
DATA_BLOCK DB3450
TITLE=
VERSION : 0.1

STRUCT
   CM_ID : STRING  [8 ] := '=PRM'; //COMPOSITE MACHINE
   STATION_ID : STRING  [8 ] := '++OP10'; //STATION - TRATTO - ZONE
   ELEMENT_ID : STRING  [8 ] := '@'; //+80FTR903
   DB_ID : INT := 1 ; //DB SIZE OR TYPE
   PART_STYLE : STRING  [12 ]; //PART STYLE ON LAST STATION
   ACT_CYCLE_TIME : INT ; //ACTUAL CYCLE TIME FOR THIS STYLE
   COUNT_GOOD : INT ; //COUNTER GOOD PIECES
   COUNT_SCRAP : INT ; //COUNTER SCRAP PIECES
   SPARE_00 : ARRAY  [0 .. 15 ] OF //SPARE INTEGER
   INT ;
   SPARE_01 : ARRAY  [0 .. 17 ] OF //SPARE INTEGER
   INT ;
   CODE_EVENT : ARRAY  [0 .. 7 ] OF //CODE EVENT - EXTENDED FAULT CODE DIAGNOSTIC
   INT ;
   EVENT : STRUCT
E0000 : BOOL ; //+80FTR903-M1; MS. SERRANDA OK;58

E0001 : BOOL ; //+80FTR903-M1; MS. APERTO;58

E0002 : BOOL ; //+80FTR903-M1; MS. CHIUSO;58

E0003 : BOOL ; //+80FTR903-M1;MS.GENERALI ERRORE;1

E0004 : BOOL ; //+80FTR903-M1; MS. MS_04;58

E0005 : BOOL ; //+80FTR903-M1; MS. MS_05;58

E0006 : BOOL ; //+80FTR903-M1; MS. MS_06;58

E0007 : BOOL ; //+80FTR903-M1; MS. MS_07;58

E0008 : BOOL ; //+80FTR903-M1; MS. MS_10;58

E0009 : BOOL ; //+80FTR903-M1; MS. MS_11;58

E0010 : BOOL ; //+80FTR903-M1; MS. MS_12;58

E0011 : BOOL ; //+80FTR903-M1; MS. MS_13;58

E0012 : BOOL ; //+80FTR903-M1; MS. MS_14;58

E0013 : BOOL ; //+80FTR903-M1; MS. MS_15;58

E0014 : BOOL ; //+80FTR903-M1; MS. MS_16;58

E0015 : BOOL ; //+80FTR903-M1; MS. MS_17;58

E0016 : BOOL ; //+80FTR903-M1; ME. DURATA APERTO;1

E0017 : BOOL ; //+80FTR903-M1; ME. DURATA CHIUDI;1

E0018 : BOOL ; //+80FTR903-M1; ME. PLAUSIBILITA;1

E0019 : BOOL ; //+80FTR903-M1; ME. FILO ROTTURA;1

E0020 : BOOL ; //+80FTR903-M1; ME. ME_04;58

E0021 : BOOL ; //+80FTR903-M1; ME. ME_05;58

E0022 : BOOL ; //+80FTR903-M1; ME. ME_06;58

E0023 : BOOL ; //+80FTR903-M1; ME. ME_07;58

E0024 : BOOL ; //+80FTR903-M1; ME. ME_10;58

E0025 : BOOL ; //+80FTR903-M1; ME. ME_11;58

E0026 : BOOL ; //+80FTR903-M1; ME. ME_12;58

E0027 : BOOL ; //+80FTR903-M1; ME. ME_13;58

E0028 : BOOL ; //+80FTR903-M1; ME. ME_14;58

E0029 : BOOL ; //+80FTR903-M1; ME. ME_15;58

E0030 : BOOL ; //+80FTR903-M1; ME. ME_16;58

E0031 : BOOL ; //+80FTR903-M1; ME. ME_17;58

E0032 : BOOL ; //+80FTR903-Y1_1; MS. APERTO;58

E0033 : BOOL ; //+80FTR903-Y1_1; MS. CHIUSO;58

E0034 : BOOL ; //+80FTR903-Y1_1;MS.GENERALI ERRORE;1

E0035 : BOOL ; //+80FTR903-Y1_1;MS.GENERALI AVVERTIMENTO;2

E0036 : BOOL ; //+80FTR903-Y1_1; MS. MS_04;58

E0037 : BOOL ; //+80FTR903-Y1_1; MS. MS_05;58

E0038 : BOOL ; //+80FTR903-Y1_1; MS. MS_06;58

E0039 : BOOL ; //+80FTR903-Y1_1; MS. MS_07;58

E0040 : BOOL ; //+80FTR903-Y1_1; MS. MS_10;58

E0041 : BOOL ; //+80FTR903-Y1_1; MS. MS_11;58

E0042 : BOOL ; //+80FTR903-Y1_1; MS. MS_12;58

E0043 : BOOL ; //+80FTR903-Y1_1; MS. MS_13;58

E0044 : BOOL ; //+80FTR903-Y1_1; MS. MS_14;58

E0045 : BOOL ; //+80FTR903-Y1_1; MS. MS_15;58

E0046 : BOOL ; //+80FTR903-Y1_1; MS. MS_16;58

E0047 : BOOL ; //+80FTR903-Y1_1; MS. MS_17;58

E0048 : BOOL ; //+80FTR903-Y1_1; ME. DURATA APERTO;1

E0049 : BOOL ; //+80FTR903-Y1_1; ME. DURATA CHIUDI;1

E0050 : BOOL ; //+80FTR903-Y1_1; ME. PLAUSIBILITA;1

E0051 : BOOL ; //+80FTR903-Y1_1; ME. FILO ROTTURA;1

E0052 : BOOL ; //+80FTR903-Y1_1; ME. PERSO POSIZIONE APERTO;2

E0053 : BOOL ; //+80FTR903-Y1_1; ME. PERSO POSIZIONE CHIUSA;2

E0054 : BOOL ; //+80FTR903-Y1_1; ME. ME_06;58

E0055 : BOOL ; //+80FTR903-Y1_1; ME. ME_07;58

E0056 : BOOL ; //+80FTR903-Y1_1; ME. ME_10;58

E0057 : BOOL ; //+80FTR903-Y1_1; ME. ME_11;58

E0058 : BOOL ; //+80FTR903-Y1_1; ME. ME_12;58

E0059 : BOOL ; //+80FTR903-Y1_1; ME. ME_13;58

E0060 : BOOL ; //+80FTR903-Y1_1; ME. ME_14;58

E0061 : BOOL ; //+80FTR903-Y1_1; ME. ME_15;58

E0062 : BOOL ; //+80FTR903-Y1_1; ME. ME_16;58

E0063 : BOOL ; //+80FTR903-Y1_1; ME. ME_17;58

E0064 : BOOL ; //+80FTR903-Y1_2; MS. APERTO;58

E0065 : BOOL ; //+80FTR903-Y1_2; MS. CHIUSO;58

E0066 : BOOL ; //+80FTR903-Y1_2;MS.GENERALI ERRORE;1

E0067 : BOOL ; //+80FTR903-Y1_2;MS.GENERALI AVVERTIMENTO;2

E0068 : BOOL ; //+80FTR903-Y1_2; MS. MS_04;58

E0069 : BOOL ; //+80FTR903-Y1_2; MS. MS_05;58

E0070 : BOOL ; //+80FTR903-Y1_2; MS. MS_06;58

E0071 : BOOL ; //+80FTR903-Y1_2; MS. MS_07;58

E0072 : BOOL ; //+80FTR903-Y1_2; MS. MS_10;58

E0073 : BOOL ; //+80FTR903-Y1_2; MS. MS_11;58

E0074 : BOOL ; //+80FTR903-Y1_2; MS. MS_12;58

E0075 : BOOL ; //+80FTR903-Y1_2; MS. MS_13;58

E0076 : BOOL ; //+80FTR903-Y1_2; MS. MS_14;58

E0077 : BOOL ; //+80FTR903-Y1_2; MS. MS_15;58

E0078 : BOOL ; //+80FTR903-Y1_2; MS. MS_16;58

E0079 : BOOL ; //+80FTR903-Y1_2; MS. MS_17;58

E0080 : BOOL ; //+80FTR903-Y1_2; ME. DURATA APERTO;1

E0081 : BOOL ; //+80FTR903-Y1_2; ME. DURATA CHIUDI;1

E0082 : BOOL ; //+80FTR903-Y1_2; ME. PLAUSIBILITA;1

E0083 : BOOL ; //+80FTR903-Y1_2; ME. FILO ROTTURA;1

E0084 : BOOL ; //+80FTR903-Y1_2; ME. PERSO POSIZIONE APERTO;2

E0085 : BOOL ; //+80FTR903-Y1_2; ME. PERSO POSIZIONE CHIUSA;2

E0086 : BOOL ; //+80FTR903-Y1_2; ME. ME_06;58

E0087 : BOOL ; //+80FTR903-Y1_2; ME. ME_07;58

E0088 : BOOL ; //+80FTR903-Y1_2; ME. ME_10;58

E0089 : BOOL ; //+80FTR903-Y1_2; ME. ME_11;58

E0090 : BOOL ; //+80FTR903-Y1_2; ME. ME_12;58

E0091 : BOOL ; //+80FTR903-Y1_2; ME. ME_13;58

E0092 : BOOL ; //+80FTR903-Y1_2; ME. ME_14;58

E0093 : BOOL ; //+80FTR903-Y1_2; ME. ME_15;58

E0094 : BOOL ; //+80FTR903-Y1_2; ME. ME_16;58

E0095 : BOOL ; //+80FTR903-Y1_2; ME. ME_17;58

E0096 : BOOL ; //+80FTR903-Y1_3; MS. APERTO;58

E0097 : BOOL ; //+80FTR903-Y1_3; MS. CHIUSO;58

E0098 : BOOL ; //+80FTR903-Y1_3;MS.GENERALI ERRORE;1

E0099 : BOOL ; //+80FTR903-Y1_3;MS.GENERALI AVVERTIMENTO;2

E0100 : BOOL ; //+80FTR903-Y1_3; MS. MS_04;58

E0101 : BOOL ; //+80FTR903-Y1_3; MS. MS_05;58

E0102 : BOOL ; //+80FTR903-Y1_3; MS. MS_06;58

E0103 : BOOL ; //+80FTR903-Y1_3; MS. MS_07;58

E0104 : BOOL ; //+80FTR903-Y1_3; MS. MS_10;58

E0105 : BOOL ; //+80FTR903-Y1_3; MS. MS_11;58

E0106 : BOOL ; //+80FTR903-Y1_3; MS. MS_12;58

E0107 : BOOL ; //+80FTR903-Y1_3; MS. MS_13;58

E0108 : BOOL ; //+80FTR903-Y1_3; MS. MS_14;58

E0109 : BOOL ; //+80FTR903-Y1_3; MS. MS_15;58

E0110 : BOOL ; //+80FTR903-Y1_3; MS. MS_16;58

E0111 : BOOL ; //+80FTR903-Y1_3; MS. MS_17;58

E0112 : BOOL ; //+80FTR903-Y1_3; ME. DURATA APERTO;1

E0113 : BOOL ; //+80FTR903-Y1_3; ME. DURATA CHIUDI;1

E0114 : BOOL ; //+80FTR903-Y1_3; ME. PLAUSIBILITA;1

E0115 : BOOL ; //+80FTR903-Y1_3; ME. FILO ROTTURA;1

E0116 : BOOL ; //+80FTR903-Y1_3; ME. PERSO POSIZIONE APERTO;2

E0117 : BOOL ; //+80FTR903-Y1_3; ME. PERSO POSIZIONE CHIUSA;2

E0118 : BOOL ; //+80FTR903-Y1_3; ME. ME_06;58

E0119 : BOOL ; //+80FTR903-Y1_3; ME. ME_07;58

E0120 : BOOL ; //+80FTR903-Y1_3; ME. ME_10;58

E0121 : BOOL ; //+80FTR903-Y1_3; ME. ME_11;58

E0122 : BOOL ; //+80FTR903-Y1_3; ME. ME_12;58

E0123 : BOOL ; //+80FTR903-Y1_3; ME. ME_13;58

E0124 : BOOL ; //+80FTR903-Y1_3; ME. ME_14;58

E0125 : BOOL ; //+80FTR903-Y1_3; ME. ME_15;58

E0126 : BOOL ; //+80FTR903-Y1_3; ME. ME_16;58

E0127 : BOOL ; //+80FTR903-Y1_3; ME. ME_17;58

E0128 : BOOL ; //+80FTR903-A1; MS. DISPLAY RILASCIATO;58

E0129 : BOOL ; //+80FTR903-A1; MS. MS_01;58

E0130 : BOOL ; //+80FTR903-A1; MS. MS_02;58

E0131 : BOOL ; //+80FTR903-A1; MS. MS_03;58

E0132 : BOOL ; //+80FTR903-A1; MS. MS_04;58

E0133 : BOOL ; //+80FTR903-A1; MS. MS_05;58

E0134 : BOOL ; //+80FTR903-A1; MS. MS_06;58

E0135 : BOOL ; //+80FTR903-A1; MS. MS_07;58

E0136 : BOOL ; //+80FTR903-A1; MS. MS_10;58

E0137 : BOOL ; //+80FTR903-A1; MS. MS_11;58

E0138 : BOOL ; //+80FTR903-A1; MS. MS_12;58

E0139 : BOOL ; //+80FTR903-A1; MS. MS_13;58

E0140 : BOOL ; //+80FTR903-A1; MS. MS_14;58

E0141 : BOOL ; //+80FTR903-A1; MS. MS_15;58

E0142 : BOOL ; //+80FTR903-A1; MS. MS_16;58

E0143 : BOOL ; //+80FTR903-A1; MS. MS_17;58

E0144 : BOOL ; //+80FTR903-A1; ME. ME_00;58

E0145 : BOOL ; //+80FTR903-A1; ME. ME_01;58

E0146 : BOOL ; //+80FTR903-A1; ME. ME_02;58

E0147 : BOOL ; //+80FTR903-A1; ME. ME_03;58

E0148 : BOOL ; //+80FTR903-A1; ME. ME_04;58

E0149 : BOOL ; //+80FTR903-A1; ME. ME_05;58

E0150 : BOOL ; //+80FTR903-A1; ME. ME_06;58

E0151 : BOOL ; //+80FTR903-A1; ME. ME_07;58

E0152 : BOOL ; //+80FTR903-A1; ME. ME_10;58

E0153 : BOOL ; //+80FTR903-A1; ME. ME_11;58

E0154 : BOOL ; //+80FTR903-A1; ME. ME_12;58

E0155 : BOOL ; //+80FTR903-A1; ME. ME_13;58

E0156 : BOOL ; //+80FTR903-A1; ME. ME_14;58

E0157 : BOOL ; //+80FTR903-A1; ME. ME_15;58

E0158 : BOOL ; //+80FTR903-A1; ME. ME_16;58

E0159 : BOOL ; //+80FTR903-A1; ME. ME_17;58

E0160 : BOOL ; //+80FTR903-A2;MS.MODO AUTOMATICO;19

E0161 : BOOL ; //+80FTR903-A2;MS.MODALITA MANUALE;16

E0162 : BOOL ; //+80FTR903-A2; MS. ECUBE A DISPOSIZIONE;58

E0163 : BOOL ; //+80FTR903-A2; MS. ECUBE NON DISPONIBILE;58

E0164 : BOOL ; //+80FTR903-A2; MS. ECUBE BLOCCATO;58

E0165 : BOOL ; //+80FTR903-A2; MS. ECUBE SBLOCCATO;58

E0166 : BOOL ; //+80FTR903-A2; MS. ECUBE ATTRACCO;58

E0167 : BOOL ; //+80FTR903-A2; MS. ECUBE ATTRACCATO;58

E0168 : BOOL ; //+80FTR903-A2; MS. ECUBE SGANCIO;58

E0169 : BOOL ; //+80FTR903-A2; MS. ECUBE SGANCIATO;58

E0170 : BOOL ; //+80FTR903-A2; MS. STAMPA ERRORE;58

E0171 : BOOL ; //+80FTR903-A2; MS. AVVIO PRODUZIONE;19

E0172 : BOOL ; //+80FTR903-A2; MS. PRODUZIONE PRONTO;19

E0173 : BOOL ; //+80FTR903-A2;MS.GENERALI ERRORE;1

E0174 : BOOL ; //+80FTR903-A2;MS.GENERALI AVVERTIMENTO;2

E0175 : BOOL ; //+80FTR903-A2;MS.RILASCIO;17

E0176 : BOOL ; //+80FTR903-A2; ME. ECUBE TIPO SBAGLIATO;1

E0177 : BOOL ; //+80FTR903-A2; ME. COMUNICAZIONE TIMEOUT;1

E0178 : BOOL ; //+80FTR903-A2; ME. SEGNALE RFID PERSO;1

E0179 : BOOL ; //+80FTR903-A2; ME. ATTRACCATO IMPOSSIBILE;1

E0180 : BOOL ; //+80FTR903-A2; ME. SGANCIATO IMPOSSIBLE;1

E0181 : BOOL ; //+80FTR903-A2; ME. ATTRACCATO FALLITO;1

E0182 : BOOL ; //+80FTR903-A2; ME. SGANCIATO FALLITO;1

E0183 : BOOL ; //+80FTR903-A2; ME. SOSTITUIRE TEMPO SCADUTO;2

E0184 : BOOL ; //+80FTR903-A2; ME. ME_10;58

E0185 : BOOL ; //+80FTR903-A2; ME. ME_11;58

E0186 : BOOL ; //+80FTR903-A2; ME. ME_12;58

E0187 : BOOL ; //+80FTR903-A2; ME. ME_13;58

E0188 : BOOL ; //+80FTR903-A2; ME. ME_14;58

E0189 : BOOL ; //+80FTR903-A2; ME. ME_15;58

E0190 : BOOL ; //+80FTR903-A2; ME. ME_16;58

E0191 : BOOL ; //+80FTR903-A2; ME. ME_17;58

E0192 : BOOL ; //+80FTR903-A3; MS. ORIFICE SENSORE DI PRESSIONE OK;58

E0193 : BOOL ; //+80FTR903-A3; MS. ORIFICE ERRORE GENERALE;1

E0194 : BOOL ; //+80FTR903-A3; MS. ORIFICE AVVERTENZE GENERALE;2

E0195 : BOOL ; //+80FTR903-A3; MS. ECUBE SENSORE DI PRESSIONE OK;58

E0196 : BOOL ; //+80FTR903-A3; MS. ECUBE ERRORE GENERALE;1

E0197 : BOOL ; //+80FTR903-A3; MS. ECEBU AVVERTENZE GENERALE;2

E0198 : BOOL ; //+80FTR903-A3; MS. 2FILTER SENSORE DI PRESSIONE OK;58

E0199 : BOOL ; //+80FTR903-A3; MS. 2FILTER ERRORE GENERALE;1

E0200 : BOOL ; //+80FTR903-A3; MS. 2FILTER AVVERTENZE GENERALE;2

E0201 : BOOL ; //+80FTR903-A3; MS. MS_11;58

E0202 : BOOL ; //+80FTR903-A3; MS. MS_12;58

E0203 : BOOL ; //+80FTR903-A3; MS. MS_13;58

E0204 : BOOL ; //+80FTR903-A3; MS. MS_14;58

E0205 : BOOL ; //+80FTR903-A3; MS. MS_15;58

E0206 : BOOL ; //+80FTR903-A3; MS. MS_16;58

E0207 : BOOL ; //+80FTR903-A3; MS. MS_17;58

E0208 : BOOL ; //+80FTR903-A3; ME. ORIFICE SONDA NON OK;1

E0209 : BOOL ; //+80FTR903-A3; ME. ORIFICE_H;2

E0210 : BOOL ; //+80FTR903-A3; ME. ORIFICE_HH;1

E0211 : BOOL ; //+80FTR903-A3; ME. ECUBE SONDA NON OK;1

E0212 : BOOL ; //+80FTR903-A3; ME. RIEMPIRE LIVELLO ECUBE_H;2

E0213 : BOOL ; //+80FTR903-A3; ME. RIEMPIRE LIVELLO ECUBE_HH;1

E0214 : BOOL ; //+80FTR903-A3; ME. 2FILTER SONDA NON OK;1

E0215 : BOOL ; //+80FTR903-A3; ME. RIEMPIRE LIVELLO 2FILTER_H;2

E0216 : BOOL ; //+80FTR903-A3; ME. RIEMPIRE LIVELLO 2FILTER_HH;1

E0217 : BOOL ; //+80FTR903-A3; ME. ME_11;58

E0218 : BOOL ; //+80FTR903-A3; ME. ME_12;58

E0219 : BOOL ; //+80FTR903-A3; ME. ME_13;58

E0220 : BOOL ; //+80FTR903-A3; ME. ME_14;58

E0221 : BOOL ; //+80FTR903-A3; ME. ME_15;58

E0222 : BOOL ; //+80FTR903-A3; ME. ME_16;58

E0223 : BOOL ; //+80FTR903-A3; ME. ME_17;58
E0224 : BOOL ;
E0225 : BOOL ;
E0226 : BOOL ;
E0227 : BOOL ;
E0228 : BOOL ;
E0229 : BOOL ;
E0230 : BOOL ;
E0231 : BOOL ;
E0232 : BOOL ;
E0233 : BOOL ;
E0234 : BOOL ;
E0235 : BOOL ;
E0236 : BOOL ;
E0237 : BOOL ;
E0238 : BOOL ;
E0239 : BOOL ;
E0240 : BOOL ;
E0241 : BOOL ;
E0242 : BOOL ;
E0243 : BOOL ;
E0244 : BOOL ;
E0245 : BOOL ;
E0246 : BOOL ;
E0247 : BOOL ;
E0248 : BOOL ;
E0249 : BOOL ;
E0250 : BOOL ;
E0251 : BOOL ;
E0252 : BOOL ;
E0253 : BOOL ;
E0254 : BOOL ;
E0255 : BOOL ;
END_STRUCT;
END_STRUCT;
BEGIN
CM_ID := '=PRM';
STATION_ID := '++OP10';
ELEMENT_ID := '@';
DB_ID := 1 ;
PART_STYLE := '';
ACT_CYCLE_TIME := 0;
COUNT_GOOD := 0;
COUNT_SCRAP := 0;
SPARE_00[0] := 0;
SPARE_00[1] := 0;
SPARE_00[2] := 0;
SPARE_00[3] := 0;
SPARE_00[4] := 0;
SPARE_00[5] := 0;
SPARE_00[6] := 0;
SPARE_00[7] := 0;
SPARE_00[8] := 0;
SPARE_00[9] := 0;
SPARE_00[10] := 0;
SPARE_00[11] := 0;
SPARE_00[12] := 0;
SPARE_00[13] := 0;
SPARE_00[14] := 0;
SPARE_00[15] := 0;
SPARE_01[0] := 0;
SPARE_01[1] := 0;
SPARE_01[2] := 0;
SPARE_01[3] := 0;
SPARE_01[4] := 0;
SPARE_01[5] := 0;
SPARE_01[6] := 0;
SPARE_01[7] := 0;
SPARE_01[8] := 0;
SPARE_01[9] := 0;
SPARE_01[10] := 0;
SPARE_01[11] := 0;
SPARE_01[12] := 0;
SPARE_01[13] := 0;
SPARE_01[14] := 0;
SPARE_01[15] := 0;
SPARE_01[16] := 0;
SPARE_01[17] := 0;
CODE_EVENT[0] := 0;
CODE_EVENT[1] := 0;
CODE_EVENT[2] := 0;
CODE_EVENT[3] := 0;
CODE_EVENT[4] := 0;
CODE_EVENT[5] := 0;
CODE_EVENT[6] := 0;
CODE_EVENT[7] := 0;
EVENT.E0000 := FALSE;
EVENT.E0001 := FALSE;
EVENT.E0002 := FALSE;
EVENT.E0003 := FALSE;
EVENT.E0004 := FALSE;
EVENT.E0005 := FALSE;
EVENT.E0006 := FALSE;
EVENT.E0007 := FALSE;
EVENT.E0008 := FALSE;
EVENT.E0009 := FALSE;
EVENT.E0010 := FALSE;
EVENT.E0011 := FALSE;
EVENT.E0012 := FALSE;
EVENT.E0013 := FALSE;
EVENT.E0014 := FALSE;
EVENT.E0015 := FALSE;
EVENT.E0016 := FALSE;
EVENT.E0017 := FALSE;
EVENT.E0018 := FALSE;
EVENT.E0019 := FALSE;
EVENT.E0020 := FALSE;
EVENT.E0021 := FALSE;
EVENT.E0022 := FALSE;
EVENT.E0023 := FALSE;
EVENT.E0024 := FALSE;
EVENT.E0025 := FALSE;
EVENT.E0026 := FALSE;
EVENT.E0027 := FALSE;
EVENT.E0028 := FALSE;
EVENT.E0029 := FALSE;
EVENT.E0030 := FALSE;
EVENT.E0031 := FALSE;
EVENT.E0032 := FALSE;
EVENT.E0033 := FALSE;
EVENT.E0034 := FALSE;
EVENT.E0035 := FALSE;
EVENT.E0036 := FALSE;
EVENT.E0037 := FALSE;
EVENT.E0038 := FALSE;
EVENT.E0039 := FALSE;
EVENT.E0040 := FALSE;
EVENT.E0041 := FALSE;
EVENT.E0042 := FALSE;
EVENT.E0043 := FALSE;
EVENT.E0044 := FALSE;
EVENT.E0045 := FALSE;
EVENT.E0046 := FALSE;
EVENT.E0047 := FALSE;
EVENT.E0048 := FALSE;
EVENT.E0049 := FALSE;
EVENT.E0050 := FALSE;
EVENT.E0051 := FALSE;
EVENT.E0052 := FALSE;
EVENT.E0053 := FALSE;
EVENT.E0054 := FALSE;
EVENT.E0055 := FALSE;
EVENT.E0056 := FALSE;
EVENT.E0057 := FALSE;
EVENT.E0058 := FALSE;
EVENT.E0059 := FALSE;
EVENT.E0060 := FALSE;
EVENT.E0061 := FALSE;
EVENT.E0062 := FALSE;
EVENT.E0063 := FALSE;
EVENT.E0064 := FALSE;
EVENT.E0065 := FALSE;
EVENT.E0066 := FALSE;
EVENT.E0067 := FALSE;
EVENT.E0068 := FALSE;
EVENT.E0069 := FALSE;
EVENT.E0070 := FALSE;
EVENT.E0071 := FALSE;
EVENT.E0072 := FALSE;
EVENT.E0073 := FALSE;
EVENT.E0074 := FALSE;
EVENT.E0075 := FALSE;
EVENT.E0076 := FALSE;
EVENT.E0077 := FALSE;
EVENT.E0078 := FALSE;
EVENT.E0079 := FALSE;
EVENT.E0080 := FALSE;
EVENT.E0081 := FALSE;
EVENT.E0082 := FALSE;
EVENT.E0083 := FALSE;
EVENT.E0084 := FALSE;
EVENT.E0085 := FALSE;
EVENT.E0086 := FALSE;
EVENT.E0087 := FALSE;
EVENT.E0088 := FALSE;
EVENT.E0089 := FALSE;
EVENT.E0090 := FALSE;
EVENT.E0091 := FALSE;
EVENT.E0092 := FALSE;
EVENT.E0093 := FALSE;
EVENT.E0094 := FALSE;
EVENT.E0095 := FALSE;
EVENT.E0096 := FALSE;
EVENT.E0097 := FALSE;
EVENT.E0098 := FALSE;
EVENT.E0099 := FALSE;
EVENT.E0100 := FALSE;
EVENT.E0101 := FALSE;
EVENT.E0102 := FALSE;
EVENT.E0103 := FALSE;
EVENT.E0104 := FALSE;
EVENT.E0105 := FALSE;
EVENT.E0106 := FALSE;
EVENT.E0107 := FALSE;
EVENT.E0108 := FALSE;
EVENT.E0109 := FALSE;
EVENT.E0110 := FALSE;
EVENT.E0111 := FALSE;
EVENT.E0112 := FALSE;
EVENT.E0113 := FALSE;
EVENT.E0114 := FALSE;
EVENT.E0115 := FALSE;
EVENT.E0116 := FALSE;
EVENT.E0117 := FALSE;
EVENT.E0118 := FALSE;
EVENT.E0119 := FALSE;
EVENT.E0120 := FALSE;
EVENT.E0121 := FALSE;
EVENT.E0122 := FALSE;
EVENT.E0123 := FALSE;
EVENT.E0124 := FALSE;
EVENT.E0125 := FALSE;
EVENT.E0126 := FALSE;
EVENT.E0127 := FALSE;
EVENT.E0128 := FALSE;
EVENT.E0129 := FALSE;
EVENT.E0130 := FALSE;
EVENT.E0131 := FALSE;
EVENT.E0132 := FALSE;
EVENT.E0133 := FALSE;
EVENT.E0134 := FALSE;
EVENT.E0135 := FALSE;
EVENT.E0136 := FALSE;
EVENT.E0137 := FALSE;
EVENT.E0138 := FALSE;
EVENT.E0139 := FALSE;
EVENT.E0140 := FALSE;
EVENT.E0141 := FALSE;
EVENT.E0142 := FALSE;
EVENT.E0143 := FALSE;
EVENT.E0144 := FALSE;
EVENT.E0145 := FALSE;
EVENT.E0146 := FALSE;
EVENT.E0147 := FALSE;
EVENT.E0148 := FALSE;
EVENT.E0149 := FALSE;
EVENT.E0150 := FALSE;
EVENT.E0151 := FALSE;
EVENT.E0152 := FALSE;
EVENT.E0153 := FALSE;
EVENT.E0154 := FALSE;
EVENT.E0155 := FALSE;
EVENT.E0156 := FALSE;
EVENT.E0157 := FALSE;
EVENT.E0158 := FALSE;
EVENT.E0159 := FALSE;
EVENT.E0160 := FALSE;
EVENT.E0161 := FALSE;
EVENT.E0162 := FALSE;
EVENT.E0163 := FALSE;
EVENT.E0164 := FALSE;
EVENT.E0165 := FALSE;
EVENT.E0166 := FALSE;
EVENT.E0167 := FALSE;
EVENT.E0168 := FALSE;
EVENT.E0169 := FALSE;
EVENT.E0170 := FALSE;
EVENT.E0171 := FALSE;
EVENT.E0172 := FALSE;
EVENT.E0173 := FALSE;
EVENT.E0174 := FALSE;
EVENT.E0175 := FALSE;
EVENT.E0176 := FALSE;
EVENT.E0177 := FALSE;
EVENT.E0178 := FALSE;
EVENT.E0179 := FALSE;
EVENT.E0180 := FALSE;
EVENT.E0181 := FALSE;
EVENT.E0182 := FALSE;
EVENT.E0183 := FALSE;
EVENT.E0184 := FALSE;
EVENT.E0185 := FALSE;
EVENT.E0186 := FALSE;
EVENT.E0187 := FALSE;
EVENT.E0188 := FALSE;
EVENT.E0189 := FALSE;
EVENT.E0190 := FALSE;
EVENT.E0191 := FALSE;
EVENT.E0192 := FALSE;
EVENT.E0193 := FALSE;
EVENT.E0194 := FALSE;
EVENT.E0195 := FALSE;
EVENT.E0196 := FALSE;
EVENT.E0197 := FALSE;
EVENT.E0198 := FALSE;
EVENT.E0199 := FALSE;
EVENT.E0200 := FALSE;
EVENT.E0201 := FALSE;
EVENT.E0202 := FALSE;
EVENT.E0203 := FALSE;
EVENT.E0204 := FALSE;
EVENT.E0205 := FALSE;
EVENT.E0206 := FALSE;
EVENT.E0207 := FALSE;
EVENT.E0208 := FALSE;
EVENT.E0209 := FALSE;
EVENT.E0210 := FALSE;
EVENT.E0211 := FALSE;
EVENT.E0212 := FALSE;
EVENT.E0213 := FALSE;
EVENT.E0214 := FALSE;
EVENT.E0215 := FALSE;
EVENT.E0216 := FALSE;
EVENT.E0217 := FALSE;
EVENT.E0218 := FALSE;
EVENT.E0219 := FALSE;
EVENT.E0220 := FALSE;
EVENT.E0221 := FALSE;
EVENT.E0222 := FALSE;
EVENT.E0223 := FALSE;
EVENT.E0224 := FALSE;
EVENT.E0225 := FALSE;
EVENT.E0226 := FALSE;
EVENT.E0227 := FALSE;
EVENT.E0228 := FALSE;
EVENT.E0229 := FALSE;
EVENT.E0230 := FALSE;
EVENT.E0231 := FALSE;
EVENT.E0232 := FALSE;
EVENT.E0233 := FALSE;
EVENT.E0234 := FALSE;
EVENT.E0235 := FALSE;
EVENT.E0236 := FALSE;
EVENT.E0237 := FALSE;
EVENT.E0238 := FALSE;
EVENT.E0239 := FALSE;
EVENT.E0240 := FALSE;
EVENT.E0241 := FALSE;
EVENT.E0242 := FALSE;
EVENT.E0243 := FALSE;
EVENT.E0244 := FALSE;
EVENT.E0245 := FALSE;
EVENT.E0246 := FALSE;
EVENT.E0247 := FALSE;
EVENT.E0248 := FALSE;
EVENT.E0249 := FALSE;
EVENT.E0250 := FALSE;
EVENT.E0251 := FALSE;
EVENT.E0252 := FALSE;
EVENT.E0253 := FALSE;
EVENT.E0254 := FALSE;
EVENT.E0255 := FALSE;
END_DATA_BLOCK
